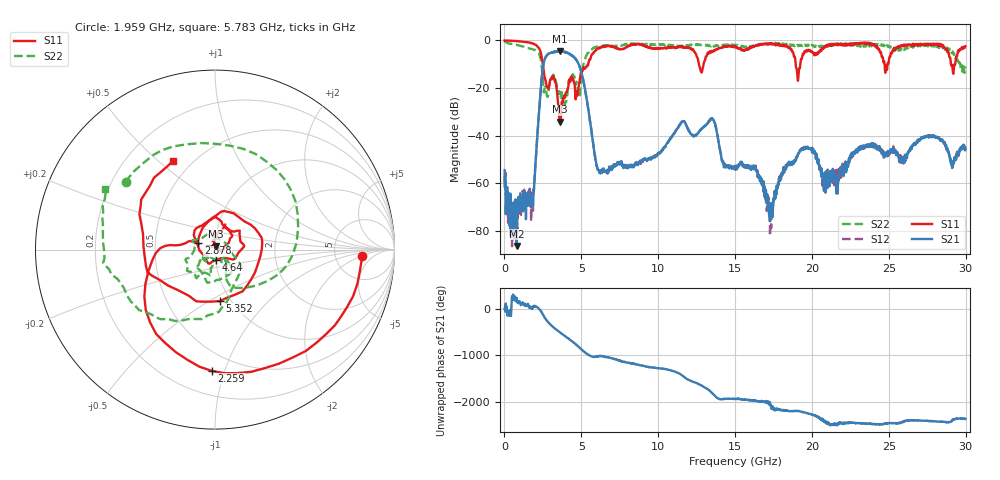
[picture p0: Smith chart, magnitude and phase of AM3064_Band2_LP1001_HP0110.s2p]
# Hz S DB R 50.0
!freq dBS11 angS11 dBS21 angS21 dBS12 angS12 dBS22 angS22
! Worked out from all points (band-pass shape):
!   1600 points, 10 MHz to 29.98 GHz, reference 50 ohm
!   highest |S21| = -4.50 dB at 3.59 GHz (marker M1); lowest = -86.4 dB at 797.2 MHz (marker M2)
!   |S21| within 3 dB of the highest: 2.646 GHz to 4.579 GHz (1.933 GHz wide, 53.5 % of centre); 4.60114 GHz to 4.602553 GHz (1.413 MHz wide, 0.0307 % of centre)
!   lowest |S11| = -34.1 dB at 3.59 GHz (marker M3), VSWR 1.04, Z = 50.5 + j1.92 ohm
!   |S11| at or under -10 dB: 2.494 GHz to 5.454 GHz (2.96 GHz wide, 74.5 % of centre); 12.64 GHz to 12.95 GHz (311.4 MHz wide, 2.43 % of centre); 18.94 GHz to 19.25 GHz (305.2 MHz wide, 1.6 % of centre)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
!   |S22| runs from -27.2 to -0.3 dB; largest |S21 - S12| = 0.017
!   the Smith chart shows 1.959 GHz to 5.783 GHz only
!   S11 on the Smith chart (normalised r, x): 1.959 GHz: 9.65, -2.21; 2.259 GHz: 0.36, -0.91; 2.878 GHz: 0.83, +0.06; 4.64 GHz: 1.00, -0.12; 5.352 GHz: 0.89, -0.56; 5.783 GHz: 0.40, +0.56
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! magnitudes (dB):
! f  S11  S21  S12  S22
! 10 MHz  0.0  -54.5  -57.1  -0.3
! 797.2 MHz  -0.3  -86.4  -68.6  -1.9
! 1.959 GHz  -1.7  -58.1  -56.9  -4.1
! 2.259 GHz  -3.4  -29.3  -29.1  -5.6
! 2.878 GHz  -20.0  -5.5  -5.6  -20.9
! 3.59 GHz  -34.1  -4.5  -4.5  -22.1
! 4.64 GHz  -24.6  -8.0  -7.8  -18.8
! 5.015 GHz  -13.0  -13.8  -13.7  -14.9
! 5.352 GHz  -10.8  -24.8  -24.7  -6.0
! 5.783 GHz  -5.2  -44.0  -44.1  -3.1
! 6.214 GHz  -3.1  -54.8  -54.2  -2.4
! 10 GHz  -3.4  -47.6  -47.4  -1.8
! 13.49 GHz  -4.4  -32.9  -32.9  -2.3
! 15 GHz  -2.6  -53.7  -53.0  -1.8
! 16.3 GHz  -2.2  -53.2  -54.0  -2.2
! 17.33 GHz  -1.3  -73.5  -68.8  -1.4
! 18.3 GHz  -2.1  -53.1  -52.4  -2.0
! 19.09 GHz  -17.0  -47.5  -48.0  -2.3
! 19.99 GHz  -4.7  -45.6  -46.2  -1.9
! 20.83 GHz  -3.0  -58.1  -55.7  -2.4
! 25 GHz  -9.1  -47.4  -47.6  -2.2
! 29.98 GHz  -2.5  -45.7  -45.2  -10.9
